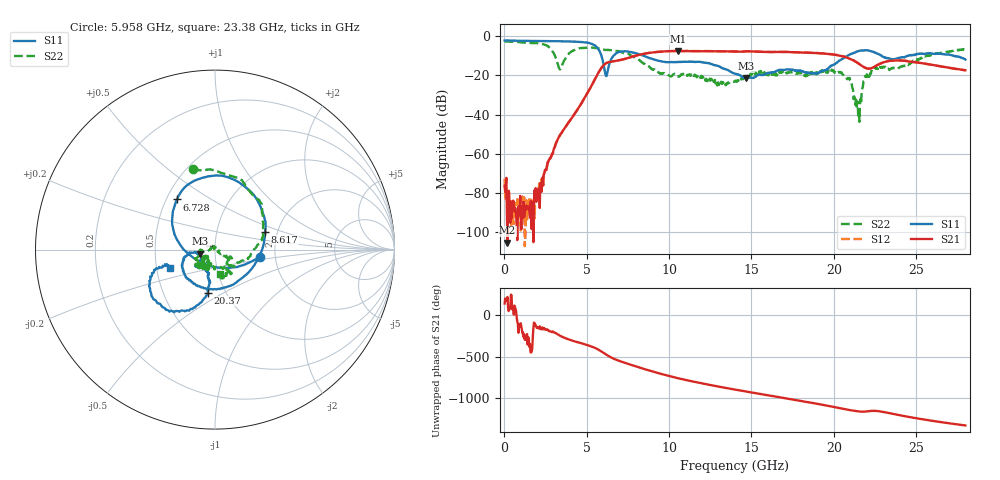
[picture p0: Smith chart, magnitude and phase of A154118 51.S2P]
!  2-Port S-parameters saved by WinCal
! VAR MeasName=S-Parameters (CALIBRATED_DATA) read from VNA (N5230A)
! VAR MeasDate=2015-9-10 14:39:06
! VAR NAME=A154118 51
! VAR FILENAME=A154118 51.S2P
! VAR DATE=2015-9-10 14:39:06
! VAR PHYS_PORTS=1,2
# Hz S DB R 50
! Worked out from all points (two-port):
!   801 points, 10 MHz to 28 GHz, reference 50 ohm
!   highest |S21| = -7.54 dB at 10.54 GHz (marker M1); lowest = -105.5 dB at 184.9 MHz (marker M2)
!   |S21| within 3 dB of the highest: 7.725 GHz to 20.67 GHz (12.94 GHz wide, 91.2 % of centre)
!   lowest |S11| = -21.4 dB at 14.67 GHz (marker M3), VSWR 1.19, Z = 42.4 - j1.86 ohm
!   |S11| at or under -10 dB: 8.472 GHz to 20.83 GHz (12.36 GHz wide, 84.4 % of centre); 22.92 GHz to 24.51 GHz (1.599 GHz wide, 6.74 % of centre); 27.29 GHz to end of sweep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
!   |S22| runs from -43.7 to -2.7 dB; largest |S21 - S12| = 0.008
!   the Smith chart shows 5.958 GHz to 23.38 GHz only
!   S11 on the Smith chart (normalised r, x): 5.958 GHz: 1.67, -0.14; 6.728 GHz: 0.57, +0.36; 8.617 GHz: 1.73, +0.38; 20.37 GHz: 0.83, -0.42; 23.38 GHz: 0.59, -0.13
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1e7  -2.15 179.7  -76.48 143.2  -72.77 -100.3  -2.67 179.8
1.849375e8  -2.16 177.2  -105.47 -137.9  -87.63 82.4  -2.70 175.5
2.10925e9  -2.43 152.1  -78.13 -161.2  -75.14 -154.4  -3.63 123.0
3.0889e9  -2.51 136.7  -55.71 147.4  -55.87 146.2  -10.39 35.9
3.613712e9  -2.62 126.6  -47.47 92.1  -47.43 92.8  -12.62 -125.2
4.698325e9  -3.01 98.2  -33.98 22.0  -33.94 22.1  -5.99 150.7
5.957875e9  -11.87 -8.9  -15.45 -84.7  -15.40 -84.6  -6.69 105.3
6.202788e9  -20.29 -122.1  -13.67 -117.4  -13.62 -117.6  -6.99 95.8
6.7276e9  -9.09 127.2  -12.64 -171.1  -12.60 -171.5  -7.52 78.2
8.616925e9  -10.53 19.6  -8.76 64.3  -8.70 64.0  -14.46 -15.5
9.351662e9  -12.53 -20.6  -7.99 21.8  -7.94 21.5  -18.57 -47.8
1.054124e10  -13.10 -83.5  -7.54 -39.0  -7.50 -39.4  -20.39 -96.0
1.4005e10  -19.14 -173.0  -7.79 -176.6  -7.76 -177.1  -23.03 -122.9
1.466976e10  -21.40 -165.2  -7.71 160.5  -7.67 160.1  -20.84 -105.0
1.869332e10  -18.75 -128.1  -8.48 22.3  -8.49 21.8  -18.24 -121.8
2.037272e10  -12.30 -99.5  -9.97 -41.0  -9.88 -41.9  -18.26 -156.6
2.10025e10  -9.27 -110.1  -11.60 -65.6  -11.49 -66.6  -22.52 -173.6
2.145734e10  -7.61 -123.1  -13.67 -79.7  -13.57 -80.9  -33.42 117.3
2.198215e10  -7.12 -141.4  -16.40 -81.1  -16.31 -82.3  -20.61 -30.8
2.334666e10  -11.41 -158.1  -12.62 -99.5  -12.61 -100.9  -16.78 -76.4
2.338165e10  -11.35 -157.8  -12.63 -100.8  -12.59 -102.2  -17.27 -79.2
2.8e10  -11.91 162.4  -17.38 110.0  -17.45 108.9  -6.45 -101.9
